ORGANIZATION_BLOCK OB 1
BEGIN
	// Test parsing of convenience operators.
	// Convenience operators are certain operators with missing white space.

	AUF	DB1
	AUF	DI1

	SET
	=	E0.1
	=	A0.1
	=	M0.1
	=	L0.1
	=	DBX0.0
	=	DIX0.0

	L	100
	T	EB0
	T	EW0
	T	ED0
	T	AB0
	T	AW0
	T	AD0
	T	LB0
	T	LW0
	T	LD0
	T	MB0
	T	MW0
	T	MD0
	T	DBB0
	T	DBW0
	T	DBD0
	T	DIB0
	T	DIW0
	T	DID0

	U	T0
	=	M0.0
	U	Z0
	=	M0.0


	CALL SFC 46 // STOP CPU
END_ORGANIZATION_BLOCK


DATA_BLOCK DB 1
STRUCT
	VARIABLE : DWORD
END_STRUCT
BEGIN
	VARIABLE := DW#16#1
END_DATA_BLOCK
